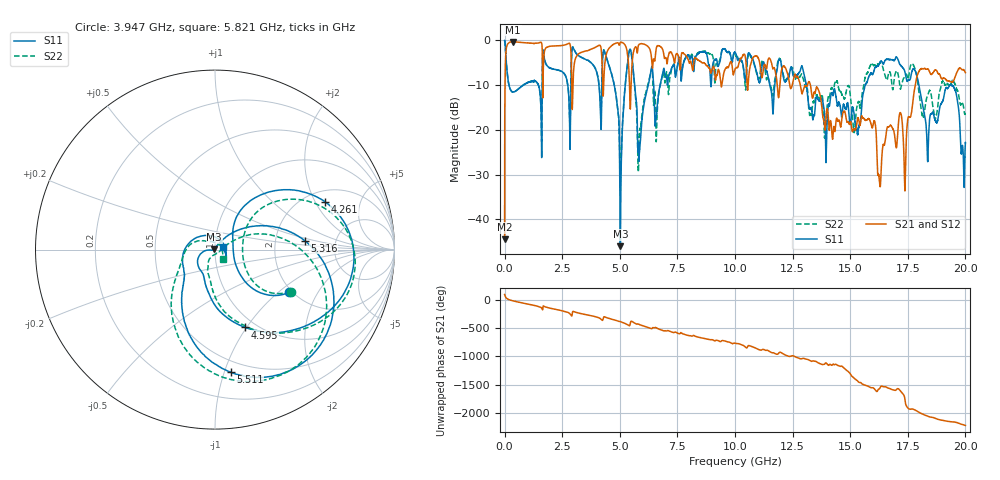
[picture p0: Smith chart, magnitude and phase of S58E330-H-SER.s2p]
!{S58E330}
!Johanson Technology Inc.
!www.johansontechnology.com
!Test Board Conditions:
!Substrate Type  RO4350B
!Substrate Thickness  60 mil
!Substrate Dk  3.66
!TL Type: GCPW
!TL Trace Width  115 mil
!TL Gap  52 mil
!Electrode orientation  Horizontal
!DUT TOPOLOGY	SERIES
!Mounting Pad LxW  55x428 mil
! Created Wed Apr 14 11:42:27 2021
# mhz S ma R 50
! 2 Port Network Data from SP1.SP block
! freq  magS11  angS11  magS21  angS21  magS12  angS12  magS22  angS22
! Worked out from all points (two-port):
!   20001 points, 300 kHz to 20 GHz, reference 50 ohm
!   highest |S21| = -0.32 dB at 373.3 MHz (marker M1); lowest = -44.5 dB at 300 kHz (marker M2)
!   |S21| within 3 dB of the highest: 47.37 MHz to 1.638 GHz (1.591 GHz wide, 189 % of centre); 1.707 GHz to 2.886 GHz (1.179 GHz wide, 51.3 % of centre)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
!   lowest |S11| = -46.0 dB at 5.023 GHz (marker M3), VSWR 1.01, Z = 49.6 + j0.238 ohm
!   |S11| at or under -10 dB: 188.7 MHz to 803.3 MHz (614.6 MHz wide, 124 % of centre); 13.09 GHz to 15.65 GHz (2.557 GHz wide, 17.8 % of centre); 17.99 GHz to 19.32 GHz (1.335 GHz wide, 7.16 % of centre)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
!   |S22| runs from -32.9 to 0.0 dB; largest |S21 - S12| = 0.0072
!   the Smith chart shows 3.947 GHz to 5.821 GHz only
!   S11 on the Smith chart (normalised r, x): 3.947 GHz: 1.93, -1.19; 4.261 GHz: 2.51, +2.42; 4.595 GHz: 0.89, -0.98; 5.316 GHz: 2.95, +0.40; 5.511 GHz: 0.40, -1.05; 5.821 GHz: 1.09, +0.03
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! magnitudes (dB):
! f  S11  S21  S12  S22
! 300 kHz  0.0  -44.5  -44.3  0.0
! 111.3 MHz  -7.2  -1.0  -1.0  -7.2
! 373.3 MHz  -11.5  -0.3  -0.3  -11.5
! 3.334 GHz  -3.8  -2.7  -2.7  -3.8
! 3.947 GHz  -6.4  -1.5  -1.5  -6.3
! 4.261 GHz  -3.5  -10.1  -10.1  -3.2
! 4.595 GHz  -6.7  -1.4  -1.4  -6.6
! 5.023 GHz  -46.0  -0.5  -0.5  -32.5
! 5.316 GHz  -6.0  -2.4  -2.4  -5.9
! 5.511 GHz  -3.2  -7.1  -7.1  -3.4
! 5.821 GHz  -26.9  -1.0  -1.0  -23.2
! 6.324 GHz  -7.7  -2.3  -2.3  -7.6
! 6.667 GHz  -12.5  -1.2  -1.2  -12.9
! 10 GHz  -2.6  -6.4  -6.4  -2.9
! 13.33 GHz  -15.8  -12.3  -12.4  -16.1
! 15.34 GHz  -20.8  -17.3  -17.3  -14.0
! 16.27 GHz  -5.3  -31.3  -31.0  -5.1
! 16.67 GHz  -4.2  -19.3  -19.5  -7.4
! 17.38 GHz  -7.2  -33.3  -33.5  -8.0
! 18.35 GHz  -25.2  -6.4  -6.5  -12.4
! 19.46 GHz  -10.2  -9.2  -9.3  -8.9
! 20 GHz  -22.9  -7.2  -7.2  -16.0
